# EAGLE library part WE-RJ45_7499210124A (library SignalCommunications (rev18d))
Order Code 7499210124A Design THT xBase-T 10/100 Base-T PoE Ports 1x1 Application PoE Tab Position UP LED (Left-Right) YELLOW-GREEN EMI Fingers No Details see: http://katalog.we-online.de/en/pbs/WE-LAN_RJ45/7499210124A? Updated by Yingchun Shan 2016-08-30 2016(C) Würth Elektronik
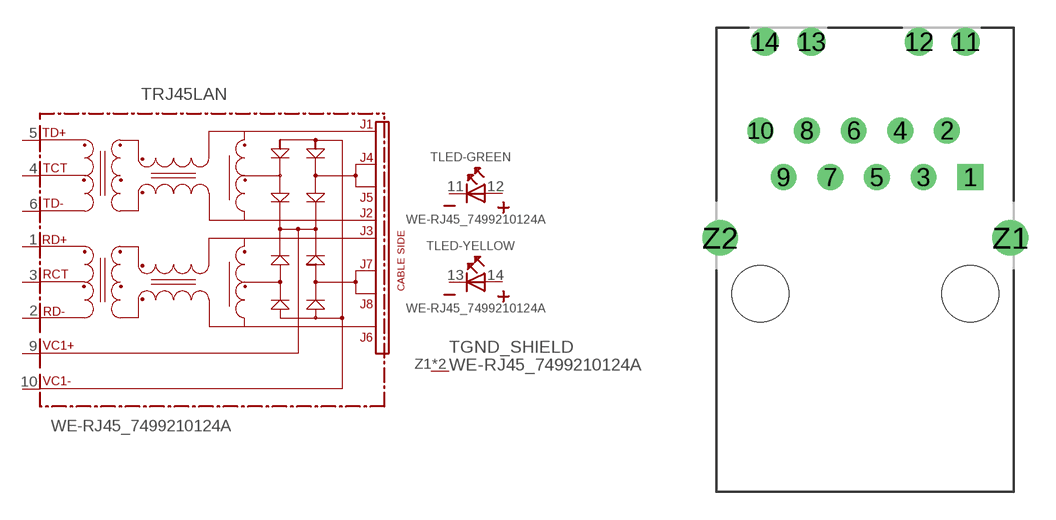
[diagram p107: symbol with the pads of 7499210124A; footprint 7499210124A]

Designator prefix T; gates RJ45LAN=749921-THT-POE-RVS LED-GREEN=LED2PIN LED-YELLOW=LED2PIN GND_SHIELD=GND_PIN

## WE-RJ45_7499210124A (COMPANY-URL: http://www.we-online.de; CREATED-BY: Christin Zierenner; CREATED-DATE: AUG 2012; DATASHEET-URL: http://katalog.we-online.de/kataloge/eisos/media/pdf/7499210124A.pdf; MANUFACTURER: Würth Elektronik eiSos GmbH)  [7499210124A]
1  RJ45LAN:RD+
2  RJ45LAN:RD-
3  RJ45LAN:RCT
4  RJ45LAN:TCT
5  RJ45LAN:TD+
6  RJ45LAN:TD-
9  RJ45LAN:VC1+  pwr
10  RJ45LAN:VC1-  pwr
11  LED-GREEN:K  pas
12  LED-GREEN:A  pas
13  LED-YELLOW:K  pas
14  LED-YELLOW:A  pas
Z1  GND_SHIELD:1  pwr
Z2  GND_SHIELD:1  pwr

## Footprint 7499210124A (pad centres in mm)
MAX HEIGHT=13.50mm PORTS----1X1 LED --YES
drill 0.9 square: 1 5.715,6.35
drill 0.9: 2 4.445,8.89; 3 3.175,6.35; 4 1.905,8.89; 5 0.635,6.35; 6 -0.635,8.89; 7 -1.905,6.35; 8 -3.175,8.89; 9 -4.445,6.35; 10 -5.715,8.89
drill 1.02: 11 5.465,13.72; 12 2.925,13.72; 13 -2.925,13.72; 14 -5.465,13.72
drill 1.3: Z1 7.9,3.05; Z2 -7.9,3.05
hole 3.1 at -5.715,0
hole 3.1 at 5.715,0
